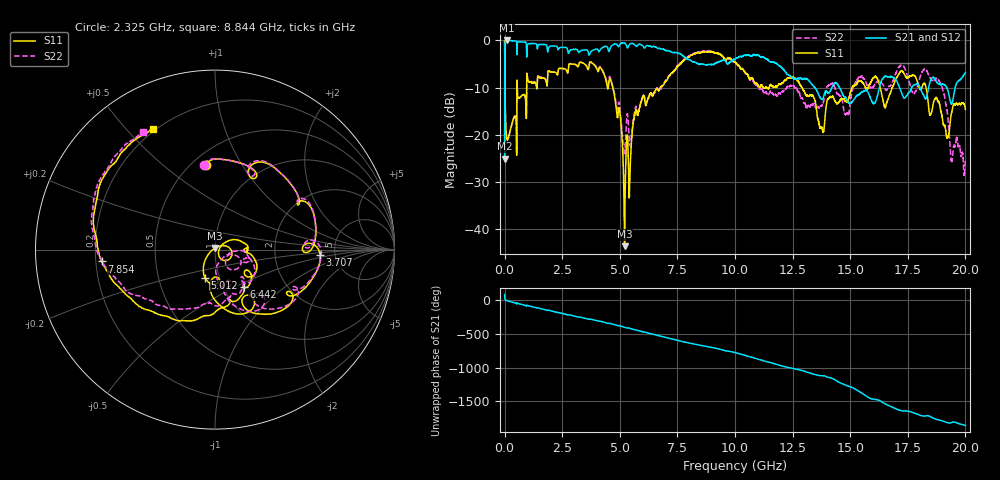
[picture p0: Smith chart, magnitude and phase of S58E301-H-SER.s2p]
!{S58E301}
!Johanson Technology Inc.
!www.johansontechnology.com
!Test Board Conditions:
!Substrate Type  RO4350B
!Substrate Thickness  60 mil
!Substrate Dk  3.66
!TL Type: GCPW
!TL Trace Width  115 mil
!TL Gap  52 mil
!Electrode orientation  Horizontal
!DUT TOPOLOGY	SERIES
!Mounting Pad LxW  55x428 mil
! Created Wed Apr 14 11:41:33 2021
# mhz S ma R 50
! 2 Port Network Data from SP1.SP block
! freq  magS11  angS11  magS21  angS21  magS12  angS12  magS22  angS22
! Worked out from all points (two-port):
!   20001 points, 300 kHz to 20 GHz, reference 50 ohm
!   highest |S21| = -0.04 dB at 86.3 MHz (marker M1); lowest = -25.0 dB at 300 kHz (marker M2)
!   |S21| within 3 dB of the highest: 965.3 MHz to 3.654 GHz (2.689 GHz wide, 116 % of centre); 3.686 GHz to 7.671 GHz (3.985 GHz wide, 70.2 % of centre)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
!   lowest |S11| = -43.5 dB at 5.206 GHz (marker M3), VSWR 1.01, Z = 49.8 + j0.62 ohm
!   |S11| at or under -10 dB: 4.695 GHz to 6.751 GHz (2.055 GHz wide, 35.9 % of centre); 12.91 GHz to 15.09 GHz (2.175 GHz wide, 15.5 % of centre); 18.29 GHz to end of sweep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
!   |S22| runs from -28.6 to -0.1 dB; largest |S21 - S12| = 0.011
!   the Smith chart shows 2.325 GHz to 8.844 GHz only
!   S11 on the Smith chart (normalised r, x): 2.325 GHz: 0.59, +0.71; 3.707 GHz: 3.80, -0.36; 5.012 GHz: 0.85, -0.28; 6.442 GHz: 1.24, -0.56; 7.854 GHz: 0.22, -0.05; 8.844 GHz: 0.19, +0.60
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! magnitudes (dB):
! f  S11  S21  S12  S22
! 300 kHz  -0.1  -25.0  -25.0  -0.1
! 86.3 MHz  -20.6  0.0  -0.1  -20.6
! 2.325 GHz  -6.5  -2.0  -2.0  -6.4
! 3.334 GHz  -4.7  -2.2  -2.2  -4.7
! 3.707 GHz  -4.6  -2.8  -2.8  -4.5
! 5.012 GHz  -15.5  -0.8  -0.8  -14.6
! 5.206 GHz  -43.5  -0.6  -0.6  -23.8
! 5.656 GHz  -15.6  -1.0  -1.0  -14.7
! 6.442 GHz  -11.6  -1.3  -1.3  -11.6
! 6.667 GHz  -10.7  -1.8  -1.8  -10.5
! 7.854 GHz  -3.9  -3.6  -3.6  -3.8
! 8.844 GHz  -2.4  -5.1  -5.2  -2.3
! 10 GHz  -4.6  -4.0  -4.0  -4.8
! 13.33 GHz  -11.6  -9.3  -9.3  -13.5
! 13.77 GHz  -18.6  -12.5  -12.4  -13.8
! 14.86 GHz  -13.0  -12.6  -12.5  -15.4
! 15.39 GHz  -8.7  -11.5  -11.5  -7.7
! 16.67 GHz  -12.1  -7.8  -7.8  -9.9
! 17.24 GHz  -6.6  -11.2  -11.2  -5.4
! 18.81 GHz  -13.0  -9.2  -9.2  -8.4
! 19.39 GHz  -15.5  -13.5  -13.4  -25.4
! 20 GHz  -14.6  -6.8  -6.8  -25.1
